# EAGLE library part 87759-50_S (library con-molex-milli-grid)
HEADER
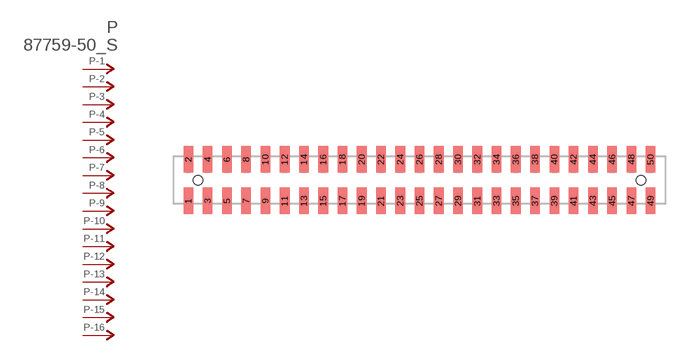
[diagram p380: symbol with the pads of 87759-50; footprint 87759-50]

Designator prefix P; gates -1=P-NV -2=P-N -3=P-N -4=P-N -5=P-N -6=P-N -7=P-N -8=P-N -9=P-N -10=P-N -11=P-N -12=P-N -13=P-N -14=P-N -15=P-N -16=P-N -17=P-N -18=P-N -19=P-N -20=P-N -21=P-N -22=P-N -23=P-N -24=P-N -25=P-N -26=P-N -27=P-N -28=P-N -29=P-N -30=P-N -31=P-N -32=P-N -33=P-N -34=P-N -35=P-N -36=P-N -37=P-N -38=P-N -39=P-N -40=P-N -41=P-N -42=P-N -43=P-N -44=P-N -45=P-N -46=P-N -47=P-N -48=P-N -49=P-N -50=P-N

## 87759-50_S  [87759-50]
1  -1:P  pas
2  -2:P  pas
3  -3:P  pas
4  -4:P  pas
5  -5:P  pas
6  -6:P  pas
7  -7:P  pas
8  -8:P  pas
9  -9:P  pas
10  -10:P  pas
11  -11:P  pas
12  -12:P  pas
13  -13:P  pas
14  -14:P  pas
15  -15:P  pas
16  -16:P  pas
17  -17:P  pas
18  -18:P  pas
19  -19:P  pas
20  -20:P  pas
21  -21:P  pas
22  -22:P  pas
23  -23:P  pas
24  -24:P  pas
25  -25:P  pas
26  -26:P  pas
27  -27:P  pas
28  -28:P  pas
29  -29:P  pas
30  -30:P  pas
31  -31:P  pas
32  -32:P  pas
33  -33:P  pas
34  -34:P  pas
35  -35:P  pas
36  -36:P  pas
37  -37:P  pas
38  -38:P  pas
39  -39:P  pas
40  -40:P  pas
41  -41:P  pas
42  -42:P  pas
43  -43:P  pas
44  -44:P  pas
45  -45:P  pas
46  -46:P  pas
47  -47:P  pas
48  -48:P  pas
49  -49:P  pas
50  -50:P  pas

## Footprint 87759-50 (pad centres in mm)
HEADER SMD Dual Row, Vertical
smd 1 x 2.75: 1 -24,-2.15; 2 -24,2.15; 3 -22,-2.15; 4 -22,2.15; 5 -20,-2.15; 6 -20,2.15; 7 -18,-2.15; 8 -18,2.15; 9 -16,-2.15; 10 -16,2.15; 11 -14,-2.15; 12 -14,2.15; 13 -12,-2.15; 14 -12,2.15; 15 -10,-2.15; 16 -10,2.15; 17 -8,-2.15; 18 -8,2.15; 19 -6,-2.15; 20 -6,2.15; 21 -4,-2.15; 22 -4,2.15; 23 -2,-2.15; 24 -2,2.15; 25 0,-2.15; 26 0,2.15; 27 2,-2.15; 28 2,2.15; 29 4,-2.15; 30 4,2.15; 31 6,-2.15; 32 6,2.15; 33 8,-2.15; 34 8,2.15; 35 10,-2.15; 36 10,2.15; 37 12,-2.15; 38 12,2.15; 39 14,-2.15; 40 14,2.15; 41 16,-2.15; 42 16,2.15; 43 18,-2.15; 44 18,2.15; 45 20,-2.15; 46 20,2.15; 47 22,-2.15; 48 22,2.15; 49 24,-2.15; 50 24,2.15
hole 1 at -23,0
hole 1 at 23,0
